(* Logix 5000 AddOnInstructionDefinition export AMCI_SD4840E2_Registration_Move_CCW; software revision 20.03 *)

ADD_ON_INSTRUCTION AMCI_SD4840E2_Registration_Move_CCW   (* revision 5.0, vendor AMCI, ExecuteEnableInFalse *)
// Revision note:
// Version 5.0 unlatches the error bit if the rung goes false.
VAR_INPUT
   Axis_Status_Bits : INT; {required}
   Type_0_for_standard_1_for_indexed : BOOL;
   Stopping_Distance : DINT; {required}
   Programmed_Speed : DINT; {required}
   Acceleration : INT; {required}
   Deceleration : INT; {required}
   Minimum_Registration_Move_Distance : DINT; {required}
END_VAR
VAR_OUTPUT
   EN : BOOL; {access Read Only, visible}
   Registration_Move_CCW_Occurring : BOOL; {access Read Only, visible}
END_VAR
VAR_IN_OUT
   AMCI_SD4840E2_output_data : _000A:SD4840E2_4342D302:O:0; {required}
END_VAR
VAR_OUTPUT
   ER : BOOL; {access Read Only, visible}
END_VAR
VAR
   Upper_Result_X_1000 : DINT;
   command_data_block : INT[10];
        [0]   // Command Bits MSW
        [1]   // Command Bits LSW
        [2]   // Upper Target Position
        [3]   // Lower Target Position
        [4]   // Upper Programmed Speed
        [5]   // Lower Programmed Speed
END_VAR

ROUTINE EnableInFalse   (* ladder *)
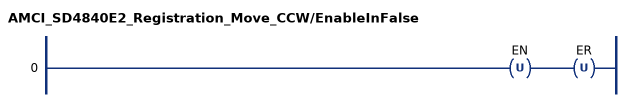
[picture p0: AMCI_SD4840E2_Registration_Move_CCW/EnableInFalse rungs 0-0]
   0: OTU(EN)OTU(ER);
END_ROUTINE

ROUTINE Logic   (* ladder *)
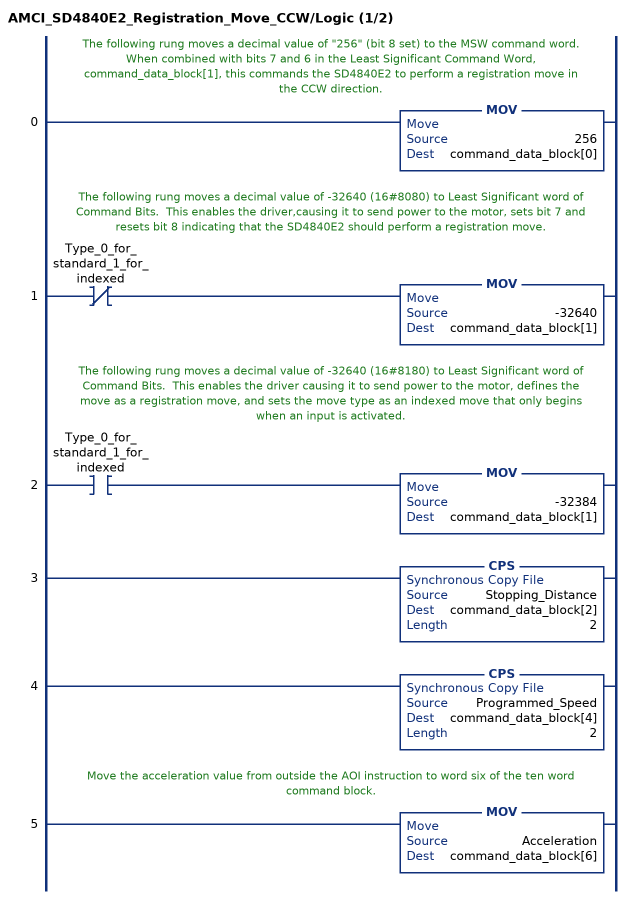
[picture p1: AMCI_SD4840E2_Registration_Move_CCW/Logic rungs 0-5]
   // The following rung moves a decimal value of "256" (bit 8 set) to the MSW command word.  When combined with bits 7 and 6 in the Least Significant Command Word, command_data_block[1], this commands the SD4840E2 to perform a registration move in the CCW direction.
   0: MOV(256,command_data_block[0]);
   // The following rung moves a decimal value of -32640 (16#8080) to Least Significant word of Command Bits.  This enables the driver,causing it to send power to the motor, sets bit 7 and resets bit 8 indicating that the SD4840E2 should perform a registration move.
   1: XIO(Type_0_for_standard_1_for_indexed)MOV(-32640,command_data_block[1]);
   // The following rung moves a decimal value of -32640 (16#8180) to Least Significant word of Command Bits.  This enables the driver causing it to send power to the motor, defines the move as a registration move, and sets the move type as an indexed move that only begins when an input is activated.
   2: XIC(Type_0_for_standard_1_for_indexed)MOV(-32384,command_data_block[1]);
   3: CPS(Stopping_Distance,command_data_block[2],2);
   4: CPS(Programmed_Speed,command_data_block[4],2);
   // Move the acceleration value from outside the AOI instruction to word six of the ten word command block.
   5: MOV(Acceleration,command_data_block[6]);
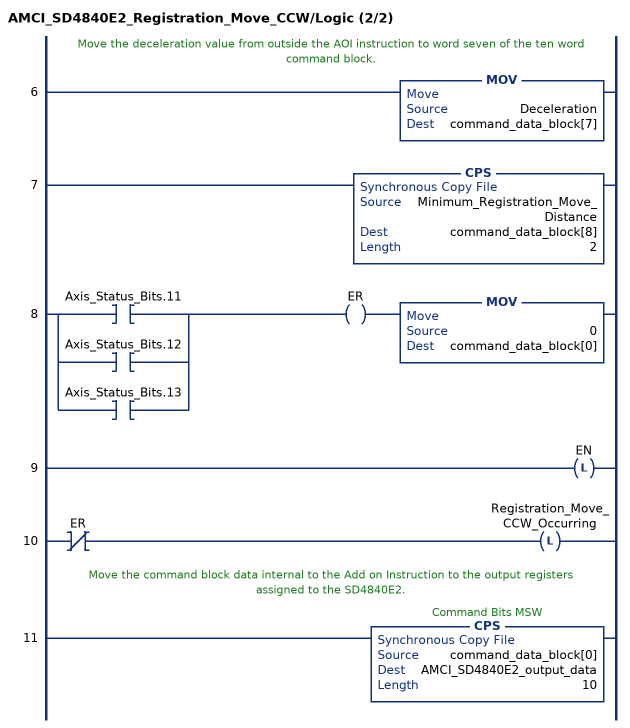
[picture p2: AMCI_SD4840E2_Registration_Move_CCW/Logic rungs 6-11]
   // Move the deceleration value from outside the AOI instruction to word seven of the ten word command block.
   6: MOV(Deceleration,command_data_block[7]);
   7: CPS(Minimum_Registration_Move_Distance,command_data_block[8],2);
   8: [XIC(Axis_Status_Bits.11) ,XIC(Axis_Status_Bits.12) ,XIC(Axis_Status_Bits.13) ]OTE(ER)MOV(0,command_data_block[0]);
   9: OTL(EN);
   10: XIO(ER)OTL(Registration_Move_CCW_Occurring);
   // Move the command block data internal to the Add on Instruction to the output registers assigned to the SD4840E2.
   11: CPS(command_data_block[0],AMCI_SD4840E2_output_data,10);
END_ROUTINE
END_ADD_ON_INSTRUCTION
